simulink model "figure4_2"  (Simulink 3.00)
settings: Solver=ode45  StartTime=0.0  StopTime=10  RelTol=1e-3

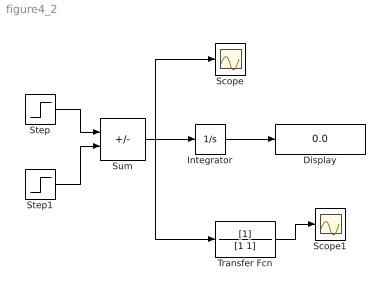
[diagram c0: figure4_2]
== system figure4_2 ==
  Display : Display
  Integrator : Integrator  ExternalReset=none  InitialConditionSource=internal  InitialCondition=0  LimitOutput=off  UpperSaturationLimit=inf  LowerSaturationLimit=-inf  ShowSaturationPort=off  ShowStatePort=off  AbsoluteTolerance=auto
  Scope : Scope
  Scope1 : Scope
  Step : Step  Time=0.50  Before=0  After=100  SampleTime=0
  Step1 : Step  Time=0.51  Before=0  After=100  SampleTime=0
  Sum : Sum  Inputs=|+-  SaturateOnIntegerOverflow=on
  Transfer Fcn : TransferFcn  Numerator=[1]  Denominator=[1 1]
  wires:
  Step/1 -> Sum/1
  Step1/1 -> Sum/2
  Integrator/1 -> Display/1
  Sum/1 -> Integrator/1, Scope/1, Transfer Fcn/1
  Transfer Fcn/1 -> Scope1/1
